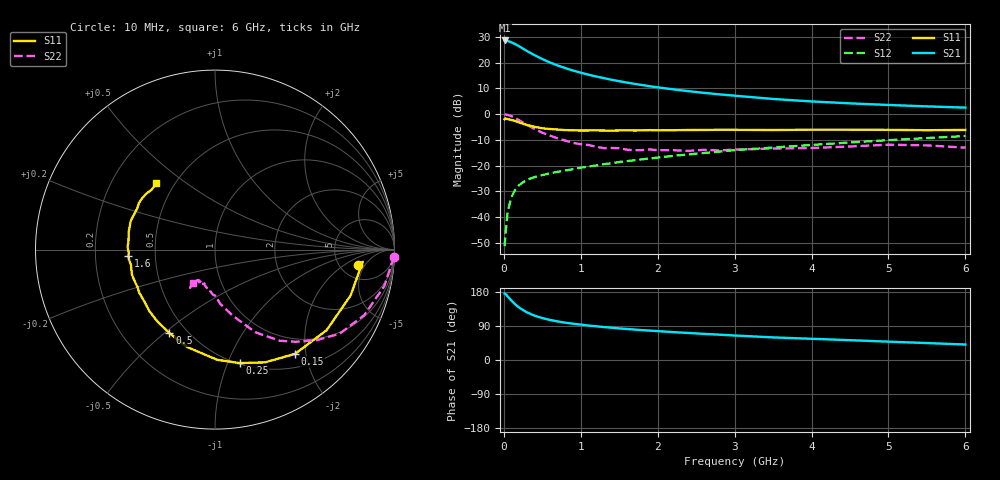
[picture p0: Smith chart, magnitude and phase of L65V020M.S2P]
!  INFINEON TECHNOLOGIES Small Signal Semiconductors
! BFR380L3 , Si-NPN RF-Transistor in TSLP-3-1
!  Vce=5 V,  Ic=20 mA
! Common Emitter S-Parameters:  07. March 2005
#  GHz  S  MA  R  50
! f  S11  S21  S12  S22
! GHz  Mag  Ang  Mag  Ang  Mag  Ang  Mag  Ang
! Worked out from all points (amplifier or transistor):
!   36 points, 10 MHz to 6 GHz, reference 50 ohm
!   highest |S21| = 28.6 dB at 10 MHz (marker M1)
!   |S21| within 3 dB of that: start of sweep to 239.8 MHz
!   unconditionally stable (mu >= 1): 2.278 GHz to 4.733 GHz
!   at 250 MHz: K = 0.30, MSG = 26.0 dB, |S12| = -26.5 dB
!   at 1.4 GHz: K = 0.91, MSG = 16.2 dB, |S12| = -19.1 dB
!   at 6 GHz: K = 0.97, MSG = 5.5 dB, |S12| = -8.5 dB
!   S11 on the Smith chart (normalised r, x): 10 MHz: 7.31, -3.43; 150 MHz: 0.72, -1.81; 250 MHz: 0.51, -1.11; 500 MHz: 0.40, -0.52; 1.6 GHz: 0.35, -0.03; 6 GHz: 0.40, +0.39
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0.01  0.7989 -6.1  27.07 175.5  0.0027 73.2  0.9993 -2.4
0.02  0.8259 -4.7  26.8 175.1  0.0044 80.0  0.9854 -5.0
0.05  0.7975 -18.7  26.4 167.7  0.0128 82.3  0.9647 -12.2
0.1  0.7671 -35.9  24.85 156.7  0.0246 73.3  0.9083 -23.7
0.15  0.7327 -52.4  22.93 146.6  0.0342 65.9  0.8379 -34.0
0.2  0.6873 -66.1  20.75 138.3  0.0416 61.4  0.7605 -41.5
0.25  0.647 -77.7  18.77 131.7  0.0473 57.6  0.6817 -48.9
0.3  0.6143 -88.8  16.9 125.8  0.0526 55.4  0.6219 -54.7
0.4  0.5649 -105.8  13.98 116.9  0.0597 52.0  0.5113 -64.1
0.5  0.5302 -118.6  11.77 110.7  0.0652 51.1  0.435 -69.5
0.6  0.5126 -129.0  10.08 105.7  0.0707 50.7  0.3818 -74.9
0.7  0.5015 -136.7  8.831 101.8  0.0754 51.4  0.3379 -79.6
0.9  0.4857 -150.5  7.022 95.7  0.0847 53.3  0.2755 -87.4
1.1  0.4813 -158.8  5.847 90.9  0.0958 54.9  0.2509 -92.8
1.4  0.4756 -169.5  4.657 85.3  0.1105 57.1  0.2196 -99.4
1.6  0.4841 -175.6  4.105 81.8  0.1219 58.2  0.2034 -106.9
2.2  0.4858 172.2  3.036 73.6  0.154 60.2  0.1987 -112.2
2.8  0.4956 161.7  2.424 66.8  0.1864 61.7  0.1962 -120.2
3.5  0.4901 152.2  1.97 59.6  0.2236 60.8  0.2138 -121.4
4.5  0.4967 145.5  1.618 52.3  0.2811 60.6  0.2346 -122.7
5.5  0.4861 136.9  1.413 44.7  0.3424 58.0  0.2464 -123.2
6  0.4922 131.5  1.338 40.9  0.3744 56.2  0.2226 -124.2
